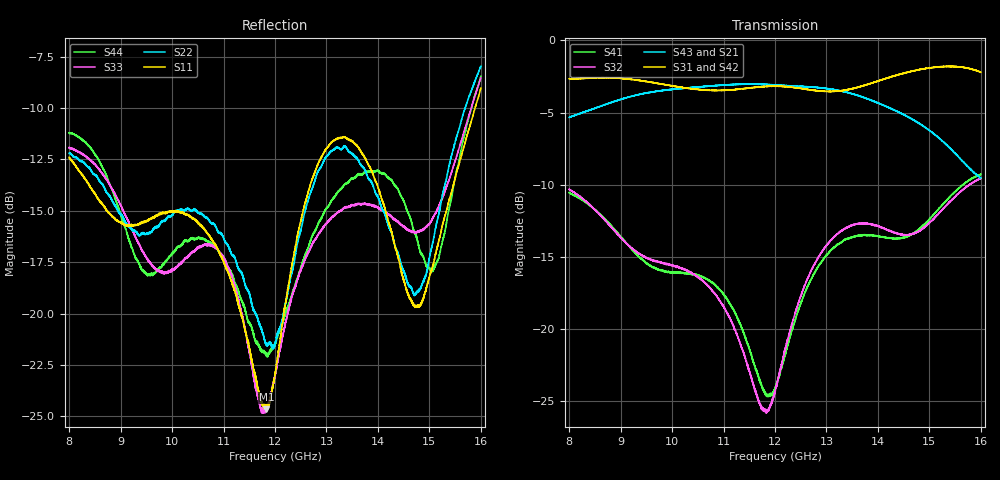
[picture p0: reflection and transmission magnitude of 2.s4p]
!Keysight Technologies,N5225A,MY51451420,A.10.40.12
!Date: Wednesday, June 29, 2016 07:51:50
!Correction: S11(Full 4 Port(1,2,3,4))
!S12(Full 4 Port(1,2,3,4))
!S13(Full 4 Port(1,2,3,4))
!S14(Full 4 Port(1,2,3,4))
!S21(Full 4 Port(1,2,3,4))
!S22(Full 4 Port(1,2,3,4))
!S23(Full 4 Port(1,2,3,4))
!S24(Full 4 Port(1,2,3,4))
!S31(Full 4 Port(1,2,3,4))
!S32(Full 4 Port(1,2,3,4))
!S33(Full 4 Port(1,2,3,4))
!S34(Full 4 Port(1,2,3,4))
!S41(Full 4 Port(1,2,3,4))
!S42(Full 4 Port(1,2,3,4))
!S43(Full 4 Port(1,2,3,4))
!S44(Full 4 Port(1,2,3,4))
!S4P File: Measurements: <S11,S12,S13,S14>,
!<S21,S22,S23,S24>,
!<S31,S32,S33,S34>,
!<S41,S42,S43,S44>:
# Hz S  dB  R 50
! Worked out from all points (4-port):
!   6401 points, 8 GHz to 16 GHz, reference 50 ohm
!   strongest paths, dB at 8 GHz, 10 GHz, 12 GHz, 14 GHz, 16 GHz:
!     S31: -2.7, -3.2, -3.2, -2.8, -2.2
!     S42: -2.7, -3.2, -3.2, -2.9, -2.4
!     S43: -5.3, -3.4, -3.1, -4.3, -9.5
!     S21: -5.2, -3.5, -3.0, -4.3, -9.5
!     S32: -10.3, -15.6, -24.4, -12.9, -9.6
!     S41: -10.6, -16.1, -24.1, -13.6, -9.3
!   lowest |S11| = -24.7 dB at 11.83 GHz (marker M1), VSWR 1.12, Z = 55.2 + j3.27 ohm
!   |S11| at or under -10 dB: start of sweep to 15.89 GHz
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8e9  -12.39 -176.5  -5.20 -117.0  -2.67 165.0  -10.57 -128.4
     -5.20 -117.0  -12.21 -154.4  -10.33 62.1  -2.69 -6.7
     -2.66 165.0  -10.33 62.1  -11.92 -155.4  -5.34 76.7
     -10.56 -128.4  -2.68 -6.8  -5.34 76.6  -11.22 -154.6
9.65375e9  -15.32 62.0  -3.64 -158.6  -2.94 115.0  -15.78 -152.6
           -3.64 -158.6  -15.82 150.2  -15.28 78.7  -2.95 -17.3
           -2.94 115.0  -15.30 78.9  -17.80 170.0  -3.55 76.3
           -15.80 -152.7  -2.96 -17.3  -3.56 76.2  -18.02 149.7
1.183375e10  -24.65 30.3  -3.02 143.8  -3.18 58.0  -24.53 75.4
             -3.02 143.7  -21.51 -133.0  -25.75 -13.5  -3.27 -22.5
             -3.20 57.9  -25.76 -13.2  -24.59 -116.0  -3.07 71.1
             -24.50 75.8  -3.27 -22.5  -3.05 71.1  -21.95 -123.5
1.3105e10  -11.66 72.0  -3.61 108.5  -3.53 23.4  -14.51 -73.0
           -3.61 108.5  -12.08 -25.8  -13.80 -119.9  -3.60 -26.8
           -3.54 23.4  -13.79 -120.0  -15.31 -13.2  -3.39 66.8
           -14.51 -73.0  -3.59 -26.9  -3.39 66.8  -14.46 -26.4
1.4495e10  -18.32 16.5  -4.93 70.2  -2.28 -14.9  -13.69 -112.1
           -4.93 70.1  -17.89 -11.9  -13.49 -131.0  -2.34 -32.2
           -2.28 -14.9  -13.49 -131.0  -15.77 -17.8  -5.14 61.2
           -13.67 -112.1  -2.34 -32.1  -5.14 61.3  -14.49 -5.5
1.50825e10  -17.52 -76.1  -6.36 53.7  -1.86 -36.3  -12.08 -114.7
            -6.36 53.7  -16.32 -78.6  -12.38 -117.1  -1.91 -39.8
            -1.87 -36.3  -12.39 -116.9  -15.30 -63.3  -6.48 60.5
            -12.10 -114.6  -1.92 -39.8  -6.46 60.4  -17.83 -60.9
1.6e10  -9.03 -174.3  -9.49 44.0  -2.20 -73.6  -9.30 -138.6
        -9.50 44.0  -7.96 -126.1  -9.57 -115.2  -2.36 -54.4
        -2.21 -73.6  -9.56 -115.3  -8.53 -115.6  -9.57 71.9
        -9.29 -138.6  -2.36 -54.5  -9.55 72.0  -8.45 -129.8
